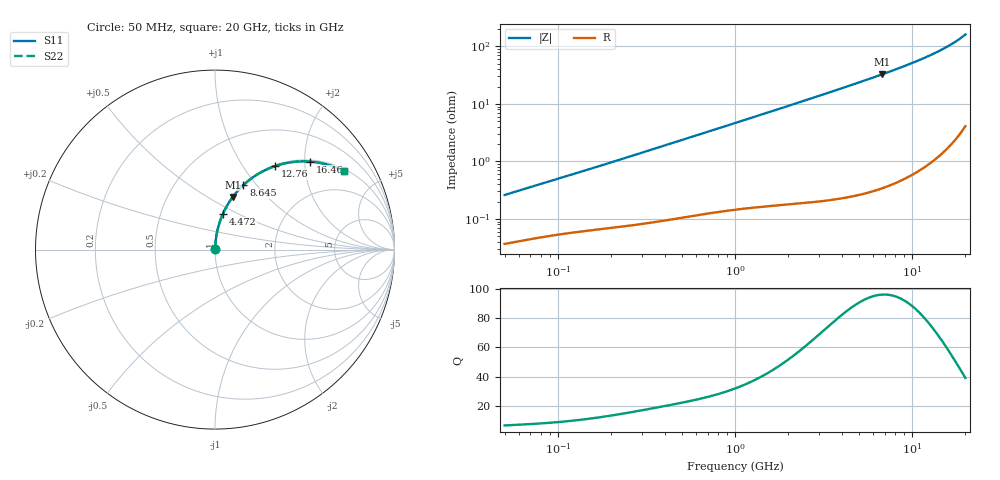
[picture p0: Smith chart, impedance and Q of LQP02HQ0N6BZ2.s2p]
!Murata Part Number: LQP02HQ0N6BZ2
!These Parameters are Measured in Series Mode Connection
!  o--[Z]--o
!Port1  Port2
!  o-------o
!Freq. Start=50[MHz] Stop=20[GHz], 401[Steps]
# Hz S RI R 50
!Freq.(Hz) S11(Real) S11(Imag) S21(Real) S21(Imag) S12(Real) S12(Imag) S22(Real) S22(Imag)
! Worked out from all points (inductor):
!   401 points, 50 MHz to 20 GHz, reference 50 ohm
!   read as one part in series: L = 808 pH near 51.52 MHz
!   highest Q = 95.8 at 6.802 GHz (marker M1), where L = 766 pH
!   S11 on the Smith chart (normalised r, x): 50 MHz: 1.00, +0.01; 4.472 GHz: 1.00, +0.42; 8.645 GHz: 1.01, +0.86; 12.76 GHz: 1.02, +1.42; 16.46 GHz: 1.04, +2.13; 20 GHz: 1.08, +3.22
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5e7  0.000374 0.00258  0.9996 -0.00258  0.9996 -0.00258  0.000374 0.00258
5.152053e7  0.00038 0.00265  0.9996 -0.00265  0.9996 -0.00265  0.00038 0.00265
1.364002e8  0.000649 0.00663  0.9994 -0.00663  0.9994 -0.00663  0.000649 0.00663
3.721004e8  0.00121 0.0175  0.9988 -0.0175  0.9988 -0.0175  0.00121 0.0175
1e9  0.00357 0.0461  0.9964 -0.0461  0.9964 -0.0461  0.00357 0.0461
1.714689e9  0.00789 0.0783  0.9921 -0.0783  0.9921 -0.0783  0.00789 0.0783
2.728004e9  0.0175 0.1236  0.9825 -0.1236  0.9825 -0.1236  0.0175 0.1236
3.519108e9  0.0279 0.1584  0.9721 -0.1584  0.9721 -0.1584  0.0279 0.1584
4.472136e9  0.044 0.1995  0.956 -0.1995  0.956 -0.1995  0.044 0.1995
5.598765e9  0.068 0.2464  0.932 -0.2464  0.932 -0.2464  0.068 0.2464
6.802353e9  0.0994 0.294  0.9006 -0.294  0.9006 -0.294  0.0994 0.294
7.442007e9  0.1185 0.318  0.8815 -0.318  0.8815 -0.318  0.1185 0.318
8.644534e9  0.1588 0.3601  0.8412 -0.3601  0.8412 -0.3601  0.1588 0.3601
9.600142e9  0.1948 0.3905  0.8052 -0.3905  0.8052 -0.3905  0.1948 0.3905
1.066139e10  0.2386 0.4204  0.7614 -0.4204  0.7614 -0.4204  0.2386 0.4204
1.166392e10  0.2835 0.4445  0.7165 -0.4445  0.7165 -0.4445  0.2835 0.4445
1.276073e10  0.336 0.4657  0.664 -0.4657  0.664 -0.4657  0.336 0.4657
1.460232e10  0.4305 0.4875  0.5695 -0.4875  0.5695 -0.4875  0.4305 0.4875
1.646126e10  0.5305 0.4902  0.4695 -0.4902  0.4695 -0.4902  0.5305 0.4902
1.800918e10  0.6141 0.4766  0.3859 -0.4766  0.3859 -0.4766  0.6141 0.4766
1.940974e10  0.6872 0.4519  0.3128 -0.4519  0.3128 -0.4519  0.6872 0.4519
2e10  0.7167 0.4381  0.2833 -0.4381  0.2833 -0.4381  0.7167 0.4381
